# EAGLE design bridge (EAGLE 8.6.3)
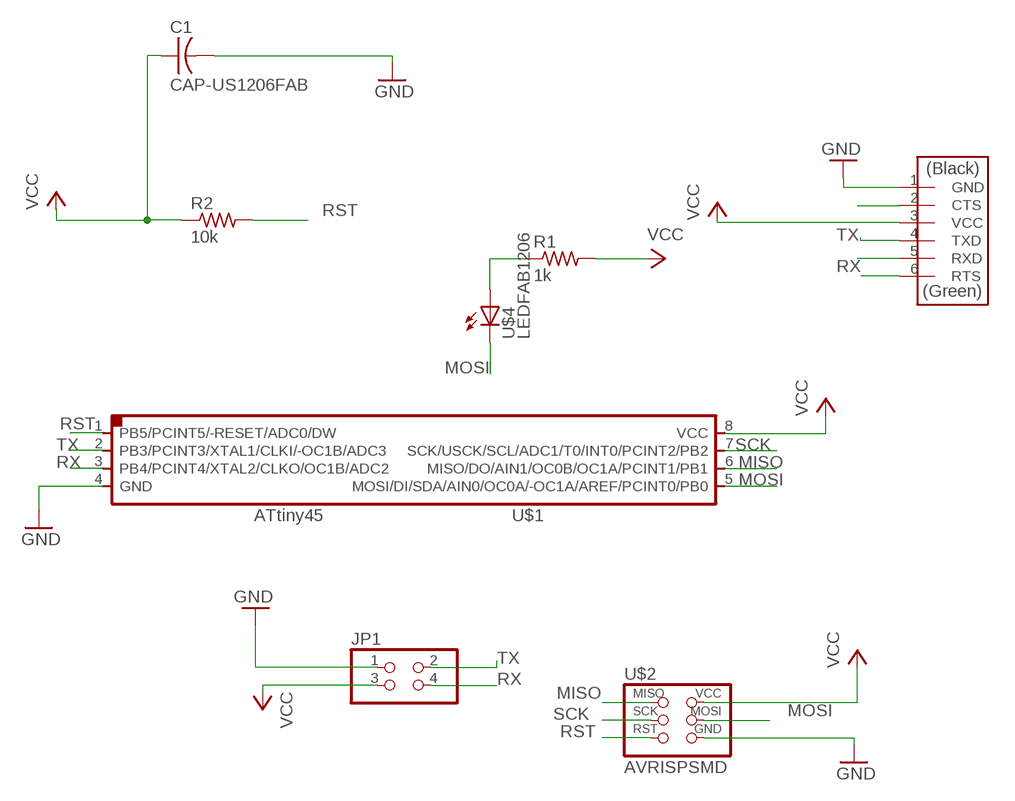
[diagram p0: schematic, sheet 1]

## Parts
C1  CAP-US1206FAB  [C1206FAB]
JP1  PINHD-2X02_2.54-SMD  [2X02SMD]
R1  1k  RES-US1206FAB  [R1206FAB]
R2  10k  RES-US1206FAB  [R1206FAB]
U$1  ATTINY45SI  [SOIC8]
U$2  AVRISPSMD  [2X03SMD]
U$3  FTDI-SMD-HEADER  [1X06SMD]
U$4  LEDFAB1206  [LED1206FAB]

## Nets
GND: C1.2 JP1.1 U$1.4(GND) U$2.6(GND) U$3.1(GND)
MISO: U$1.6(MISO/DO/AIN1/OC0B/OC1A/PCINT1/PB1) U$2.1(MISO)
MOSI: U$1.5(MOSI/DI/SDA/AIN0/OC0A/-OC1A/AREF/PCINT0/PB0) U$2.4(MOSI) U$4.2(C)
N$1: R1.1 U$4.1(A)
N$20: U$3.2(CTS)
N$24: U$3.6(RTS)
RST: R2.2 U$1.1(PB5/PCINT5/-RESET/ADC0/DW) U$2.5(RST)
RX: JP1.4 U$1.3(PB4/PCINT4/XTAL2/CLKO/OC1B/ADC2) U$3.5(RXD)
SCK: U$1.7(SCK/USCK/SCL/ADC1/T0/INT0/PCINT2/PB2) U$2.3(SCK)
TX: JP1.2 U$1.2(PB3/PCINT3/XTAL1/CLKI/-OC1B/ADC3) U$3.4(TXD)
VCC: C1.1 JP1.3 R1.2 R2.1 U$1.8(VCC) U$2.2(VCC) U$3.3(VCC)

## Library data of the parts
C1 = fab:CAP-US
JP1 = pinhead-2:PINHD-2X02: PIN HEADER
R1 R2 = fab:RES-US: Resistor (US Symbol)
U$1 = fab:ATTINY45
U$2 = fab:AVRISP
U$3 = fab:FTDI-SMD-HEADER
U$4 = fab:LED: LED

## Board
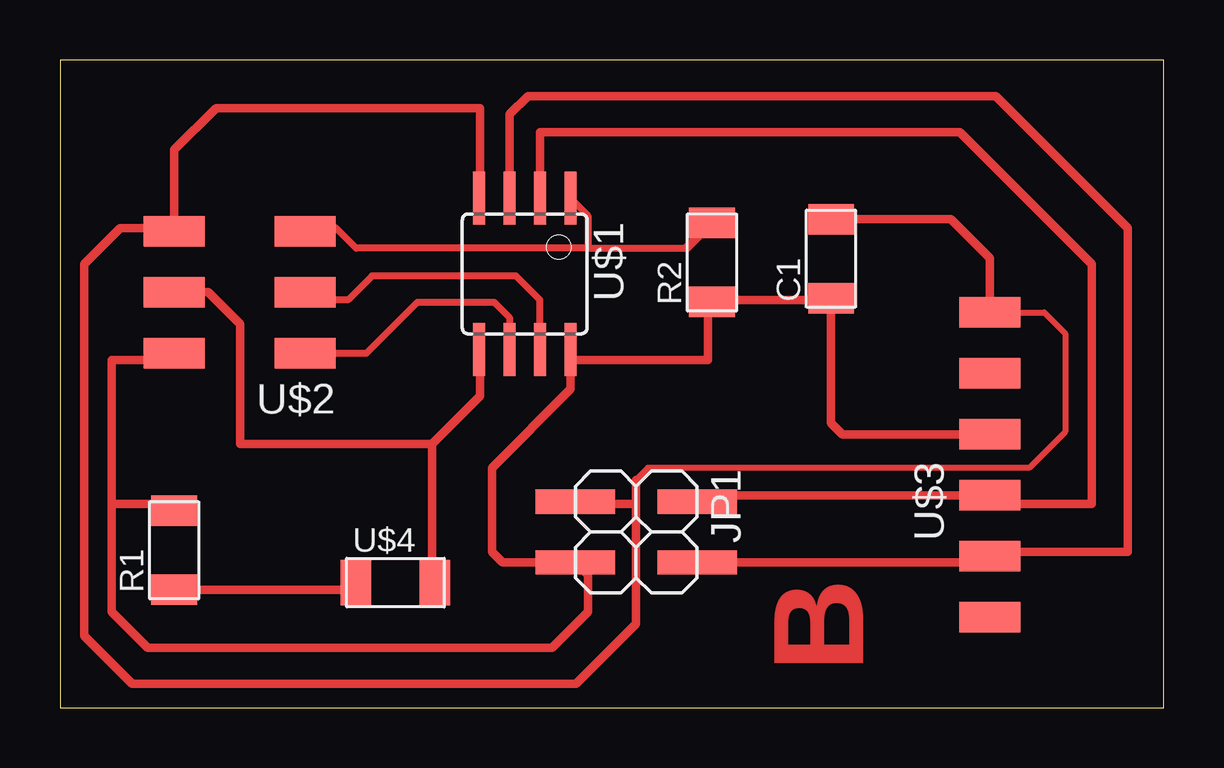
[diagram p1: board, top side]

Size 46 x 27 mm. Coordinates in mm from the lower left corner, seen from the top.
Outline: 0,0 46,0 46,27 0,27 0,0
Copper layers (1*16): Top 0.035mm / dielectric 1.5mm / Bottom 0.035mm
Design rules "default *": minimum track width 0.3mm, minimum drill 0.35mm, track to track 0.8mm, track to pad 6mil, pad to pad 6mil, via to via 6mil, smd to smd 6mil, copper to edge 0.8mm, drill to drill 6mil, minimum pad ring 10mil, minimum via ring 8mil, stop-mask expansion 4mil, vias tented up to drill 0mil, thermal gap 10mil

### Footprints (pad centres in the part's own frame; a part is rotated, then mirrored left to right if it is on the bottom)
C1206FAB = smd 1.27 x 1.905: 1 -1.651,0; 2 1.651,0
2X02SMD = smd 1.016 x 3.302: 1 -1.27,-3.81; 2 -1.27,1.27; 3 1.27,-3.81; 4 1.27,1.27
R1206FAB = smd 1.27 x 1.905: 1 -1.651,0; 2 1.651,0
SOIC8 = smd 0.5 x 2.2: 1 -1.905,-3.154; 2 -0.645,-3.154; 3 0.625,-3.154; 4 1.895,-3.154; 5 1.905,3.154; 6 0.635,3.154; 7 -0.635,3.154; 8 -1.905,3.154
2X03SMD = smd 2.54 x 1.27: 1 -2.54,2.54; 2 2.92,2.54; 3 -2.54,0; 4 2.92,0; 5 -2.54,-2.54; 6 2.92,-2.54
1X06SMD = smd 2.54 x 1.27: 1 0,6.35; 2 0,3.81; 3 0,1.27; 4 0,-1.27; 5 0,-3.81; 6 0,-6.35
LED1206FAB = smd 1.27 x 1.905: 1 -1.651,0; 2 1.651,0

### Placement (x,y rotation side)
C1  32.14,18.71 90 top
JP1  25.29,7.32 270 top
R1  4.76,6.56 90 top
R2  27.18,18.56 90 top
U$1  19.37,18.08 180 top
U$2  7.68,17.32 180 top
U$3  38.76,10.12 0 top
U$4  13.98,5.21 0 top

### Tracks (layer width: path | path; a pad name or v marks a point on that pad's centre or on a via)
GND
  Top 0.25: U$3.1 41.03,16.47 41.9,15.6 41.9,11.5 40.4,10 24.5,10 24,9.5
  Top 0.35: U$1.4 17.5,21.26 17.5,25 6.5,25 4.76,23.26 U$2.6 4.62,20 2.5,20 1,18.5 1,3 3,1 21.5,1 24,3.5 24,8.5 | C1.2 37.14,20.36 38.76,18.74 U$3.1 | 24,9.5 24,8.5 | JP1.1 21.57,8.5 24,8.5
MISO
  Top 0.3: 10.5,14.5 U$2.1 12.78,14.78 14.9,16.9 18.1,16.9 18.73,16.27 U$1.6
MOSI
  Top 0.35: U$4.2 15.5,5.34 15.5,11 | 15.5,11 17.5,13 17.5,14.89 U$1.5 | 15.5,11 7.5,11 7.5,16 6.18,17.32 U$2.4
N$1
  Top 0.35: R1.1 12.03,4.91 U$4.1
RST
  Top 0.3: 22,19.15 26.12,19.15 | U$1.1 22,20.51 22,19.15 | 22,19.15 12.35,19.15 11.5,20 10.36,20 U$2.5
  Top 0.35: 26.12,19.15 R2.2
RX
  Top 0.35: JP1.4 38.5,6.05 U$3.5 38.95,6.5 44.5,6.5 44.5,20 39,25.5 19.5,25.5 18.75,24.75 U$1.3
SCK
  Top 0.3: U$1.7 20,17 19,18 13,18 12,17 10.54,17 U$2.3
  Top 0.35: U$1.7
TX
  Top 0.35: U$1.2 20.02,23.98 20,24 37.5,24 43,18.5 43,8.5 39.11,8.5 U$3.4 26.82,8.85 JP1.2
VCC
  Top 0.35: U$2.2 4.48,14.5 2.15,14.5 2.15,8.5 | 2.15,8.5 2.15,4 3.65,2.5 20.5,2.5 22,4 22,5.53 JP1.3 18.45,6.05 18,6.5 18,10 21.27,13.28 21.27,14.5 | U$1.8 21.27,14.5 | 21.27,14.5 27,14.5 27,16.73 R2.1 27.27,17 32.14,17 | U$3.3 32.61,11.39 32.14,11.86 32.14,17 | 32.14,17 C1.1 | 2.15,8.5 4.47,8.5 R1.2

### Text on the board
Top: B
